(* Logix 5000 AddOnInstructionDefinition export YAI_Assy_166_116_EIP_Hz; software revision 21.03 *)

ADD_ON_INSTRUCTION YAI_Assy_166_116_EIP_Hz   (* revision 1.1, vendor Yaskawa America, Inc. *)
// YAI Assembly 166 and 116
// Revision note:
// Corrected Custom_Out_x function.
// Help:
// This add-on instruction is for use with input assemblie 166 and output assemblies 116.
// Node_Input_Assy is defined as the node's input assembly integer array.
// Node_Output_Assy is defined as the node's output assembly integer array.
// Torque limit/reference, torque compensation and torque output variables are only available with A1000.
VAR_IN_OUT
   Node_Input_Assy : AB:ETHERNET_MODULE_INT_44Bytes:I:0; {required}   // Input assembly words
   Node_Output_Assy : AB:ETHERNET_MODULE_INT_44Bytes:O:0; {required}   // Output assembly words
END_VAR
VAR_INPUT
   RunFwd : BOOL; {visible}   // Forward run command
   RunRev : BOOL; {visible}   // Reverse run command
   MFI_3 : BOOL; {visible}   // Multi-function input 3
   MFI_4 : BOOL; {visible}   // Multi-function input 4
   MFI_5 : BOOL; {visible}   // Multi-function input 5
   MFI_6 : BOOL; {visible}   // Multi-function input 6
   MFI_7 : BOOL; {visible}   // Multi-function input 7
   MFI_8 : BOOL; {visible}   // Multi-function input 8
   External_Fault : BOOL;   // External fault command (EF0)
   FaultReset : BOOL; {visible}   // Fault reset command
   MFO_1 : BOOL; {visible}   // Multi-function output (M1-M2 for A/P1000, MA/MB/MC for V1000)
   MFO_2 : BOOL; {visible}   // Multi-function output (M3-M4 for A/P1000, P1 for V1000)
   MFO_3 : BOOL; {visible}   // Multi-function output (M5-M6 for A/P1000, P2 for V1000)
   Freq_Ref : REAL; {visible}   // Frequency reference command in Hz (xx.xx resolution)
   Torq_Ref_Limit : REAL; {visible}   // Torque reference/limit (A1000 only)
   Torq_Comp : REAL; {visible}   // Torque compensation command (A1000 only)
   Net_Ref : BOOL;   // Network reference control bit
   Net_Control : BOOL;   // Network start/stop control bit
   Analog_Output_1 : REAL;   // Analog output 1 level command
   Analog_Output_2 : REAL;   // Analog output 2 level command
   Digital_Output_1 : BOOL;   // Digital output 1 activation - M1-M2
   Digital_Output_2 : BOOL;   // Digital output 2 activation - M3-M4
   Digital_Output_3 : BOOL;   // Digital output 3 activation - M5-M6
   Digital_Output_Fault_Enable : BOOL;   // Bit to enable control of fault output relay over the network
   Digital_Output_Fault : BOOL;   // Fault relay activation - MA-MB-MC
   Custom_Out_1 : INT; {visible}   // Custom output 1 - F7-23
   Custom_Out_2 : INT; {visible}   // Custom output 2 - F7-24
   Custom_Out_3 : INT; {visible}   // Custom output 3 - F7-25
   Custom_Out_4 : INT;   // Custom output 4 - F7-26
   Custom_Out_5 : INT;   // Custom output 5 - F7-27
   Custom_Out_6 : INT;   // Custom output 6 - F7-28
   Custom_Out_7 : INT;   // Custom output 7 - F7-29
   Custom_Out_8 : INT;   // Custom output 8 - F7-30
   Custom_Out_9 : INT;   // Custom output 9 - F7-31
   Custom_Out_10 : INT;   // Custom output 10 - F7-32
END_VAR
VAR_OUTPUT
   Running : BOOL; {access Read Only, visible}   // Drive running forward status bit
   ZSP : BOOL; {access Read Only, visible}   // Drive zero speed status bit
   RunningRev : BOOL; {access Read Only, visible}   // Drive running reverse status bit
   Reset : BOOL; {access Read Only, visible}   // Drive reset command status bit
   At_Speed : BOOL; {access Read Only, visible}   // Drive at commanded speed status bit
   Ready : BOOL; {access Read Only, visible}   // Drive ready status bit
   Alarm : BOOL; {access Read Only, visible}   // Drive alarm status bit
   Faulted : BOOL; {access Read Only, visible}   // Drive faulted status bit
   OPE : BOOL; {access Read Only}   // OPE alarm/fault present
   UV : BOOL; {access Read Only}   // Drive in UV (undervoltage) state status bit
   NetCtrlStatus : BOOL; {access Read Only, visible}   // Drive network run source status bit (1 = source coming from network)
   MFO_1_Status : BOOL; {access Read Only, visible}   // Drive multi-function output 1 (M1-M2 for A/P1000, MA/MB/MC for V1000) status
   MFO_2_Status : BOOL; {access Read Only, visible}   // Drive multi-function output 1 (M3-M4 for A/P1000, P1 for V1000) status
   MFO_3_Status : BOOL; {access Read Only, visible}   // Drive multi-function output 1 (M5-M6 for A/P1000, P2 for V1000) status
   ZSV : BOOL; {access Read Only, visible}   // Drive zero servo completed status bit
   Motor_Speed : REAL; {access Read Only, visible}   // Motor speed in Hz (xx.xx resolution)
   Torque_Actual : REAL; {access Read Only, visible}   // Drive torque output in % (xxx.x resolution)
   PG_Count : INT; {access Read Only}   // Encoder feedback count
   Freq_Cmd : REAL; {access Read Only, visible}   // Commanded frequency in Hz (xx.xx resolution)
   Output_Freq : REAL; {access Read Only, visible}   // Drive output frequency in Hz (xx.xx resolution)
   Output_Current : REAL; {access Read Only, visible}   // Drive output current in A (xxx.x resolution)
   Analog_Input_1_Level : REAL; {access Read Only}   // Analog input 1 level in % (xxx.x resolution)
   DC_Bus_Volt : INT; {access Read Only, visible}   // DC bus voltage in Vdc (xxx resolution)
   Error_Code : INT; {access Read Only}   // Custom input/output error code. Refer to custom error bit to determine which parameter error is pertaining to.
   Custom_In_1 : INT; {access Read Only, visible}   // Custom input 1 - F7-33
   Custom_In_2 : INT; {access Read Only, visible}   // Custom input 2 - F7-34
   Custom_In_3 : INT; {access Read Only, visible}   // Custom input 3 - F7-35
   Custom_In_4 : INT; {access Read Only}   // Custom input 4 - F7-36
   Custom_In_5 : INT; {access Read Only}   // Custom input 5 - F7-37
   Custom_In_6 : INT; {access Read Only}   // Custom input 6 - F7-38
   Custom_In_7 : INT; {access Read Only}   // Custom input 7 - F7-39
   Custom_In_8 : INT; {access Read Only}   // Custom input 8 -F7-40
   Custom_In_9 : INT; {access Read Only}   // Custom input 9 - F7-41
   Custom_In_10 : INT; {access Read Only}   // Custom input 10 - F7-42
   Custom_Out_1_Error : BOOL; {access Read Only}   // Custom output 1 error bit
   Custom_Out_2_Error : BOOL; {access Read Only}   // Custom output 2 error bit
   Custom_Out_3_Error : BOOL; {access Read Only}   // Custom output 3 error bit
   Custom_Out_4_Error : BOOL; {access Read Only}   // Custom output 4 error bit
   Custom_Out_5_Error : BOOL; {access Read Only}   // Custom output 5 error bit
   Custom_Out_6_Error : BOOL; {access Read Only}   // Custom output 6 error bit
   Custom_Out_7_Error : BOOL; {access Read Only}   // Custom output 7 error bit
   Custom_Out_8_Error : BOOL; {access Read Only}   // Custom output 8 error bit
   Custom_Out_9_Error : BOOL; {access Read Only}   // Custom output 9 error bit
   Custom_Out_10_Error : BOOL; {access Read Only}   // Custom output 10 error bit
   Custom_In_1_Error : BOOL; {access Read Only}   // Custom input 1 error bit
   Custom_In_2_Error : BOOL; {access Read Only}   // Custom input 2 error bit
   Custom_In_3_Error : BOOL; {access Read Only}   // Custom input 3 error bit
   Custom_In_4_Error : BOOL; {access Read Only}   // Custom input 4 error bit
   Custom_In_5_Error : BOOL; {access Read Only}   // Custom input 5 error bit
   Custom_In_6_Error : BOOL; {access Read Only}   // Custom input 6 error bit
   Custom_In_7_Error : BOOL; {access Read Only}   // Custom input 7 error bit
   Custom_In_8_Error : BOOL; {access Read Only}   // Custom input 8 error bit
   Custom_In_9_Error : BOOL; {access Read Only}   // Custom input 9 error bit
   Custom_In_10_Error : BOOL; {access Read Only}   // Custom input 10 error bit
END_VAR
VAR
   FRef_Convert : DINT;
   FOut_Convert : REAL;
   FOut_Temp : REAL;
   TRef_Convert : INT;
   TComp_Convert : INT;
   TOut_Convert : REAL;
   TOut_Temp : REAL;
   IOut_Temp : REAL;
   IOut_Convert : REAL;
   AO1_Convert : INT;
   AO2_Convert : INT;
   Motor_Speed_Temp : REAL;
   Motor_Speed_Convert : REAL;
   Freq_Cmd_Temp : REAL;
   Freq_Cmd_Convert : REAL;
   AI1_Temp : REAL;
   AI1_Convert : REAL;
END_VAR

ROUTINE Logic   (* ladder *)
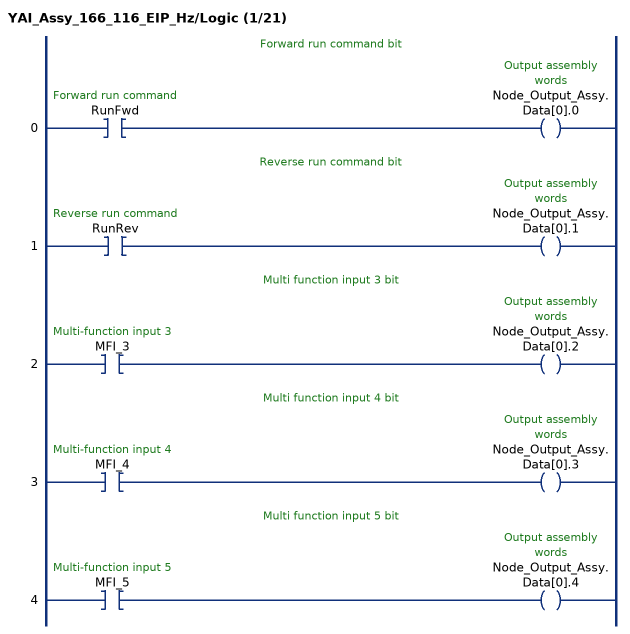
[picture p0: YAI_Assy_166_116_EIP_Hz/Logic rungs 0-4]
   // Forward run command bit
   0: XIC(RunFwd)OTE(Node_Output_Assy.Data[0].0);
   // Reverse run command bit
   1: XIC(RunRev)OTE(Node_Output_Assy.Data[0].1);
   // Multi function input 3 bit
   2: XIC(MFI_3)OTE(Node_Output_Assy.Data[0].2);
   // Multi function input 4 bit
   3: XIC(MFI_4)OTE(Node_Output_Assy.Data[0].3);
   // Multi function input 5 bit
   4: XIC(MFI_5)OTE(Node_Output_Assy.Data[0].4);
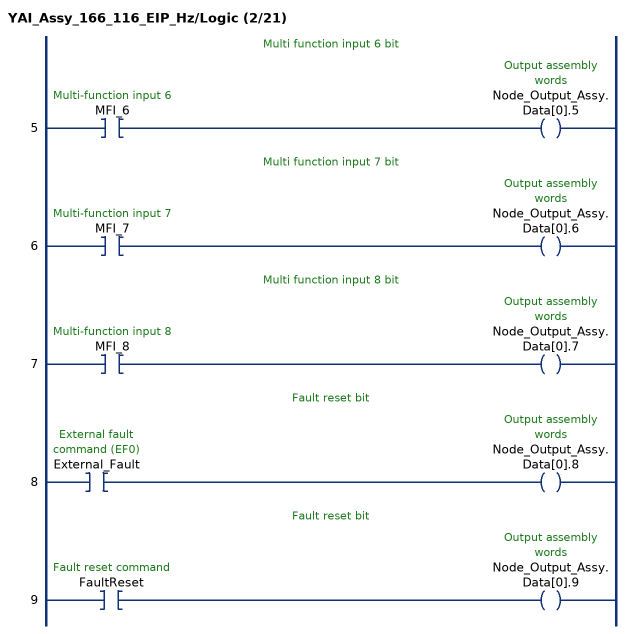
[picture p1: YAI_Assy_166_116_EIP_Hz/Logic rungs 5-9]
   // Multi function input 6 bit
   5: XIC(MFI_6)OTE(Node_Output_Assy.Data[0].5);
   // Multi function input 7 bit
   6: XIC(MFI_7)OTE(Node_Output_Assy.Data[0].6);
   // Multi function input 8 bit
   7: XIC(MFI_8)OTE(Node_Output_Assy.Data[0].7);
   // Fault reset bit
   8: XIC(External_Fault)OTE(Node_Output_Assy.Data[0].8);
   // Fault reset bit
   9: XIC(FaultReset)OTE(Node_Output_Assy.Data[0].9);
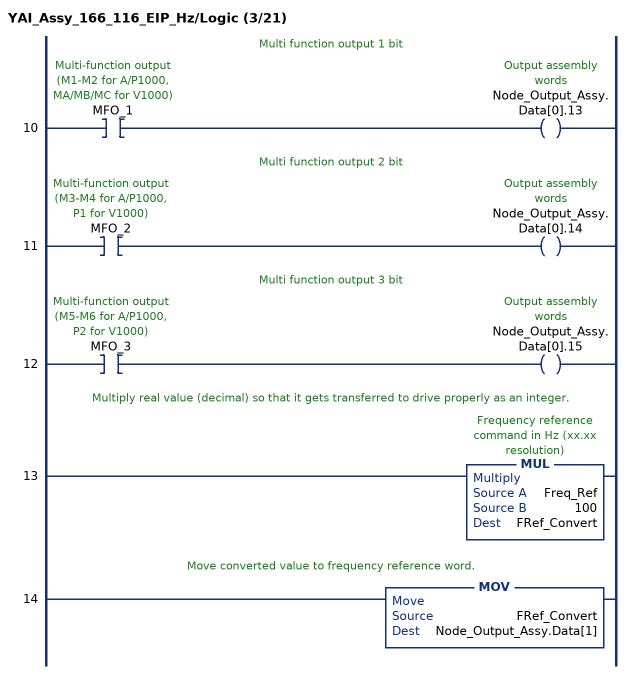
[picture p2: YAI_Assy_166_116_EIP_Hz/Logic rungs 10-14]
   // Multi function output 1 bit
   10: XIC(MFO_1)OTE(Node_Output_Assy.Data[0].13);
   // Multi function output 2 bit
   11: XIC(MFO_2)OTE(Node_Output_Assy.Data[0].14);
   // Multi function output 3 bit
   12: XIC(MFO_3)OTE(Node_Output_Assy.Data[0].15);
   // Multiply real value (decimal) so that it gets transferred to drive properly as an integer.
   13: MUL(Freq_Ref,100,FRef_Convert);
   // Move converted value to frequency reference word.
   14: MOV(FRef_Convert,Node_Output_Assy.Data[1]);
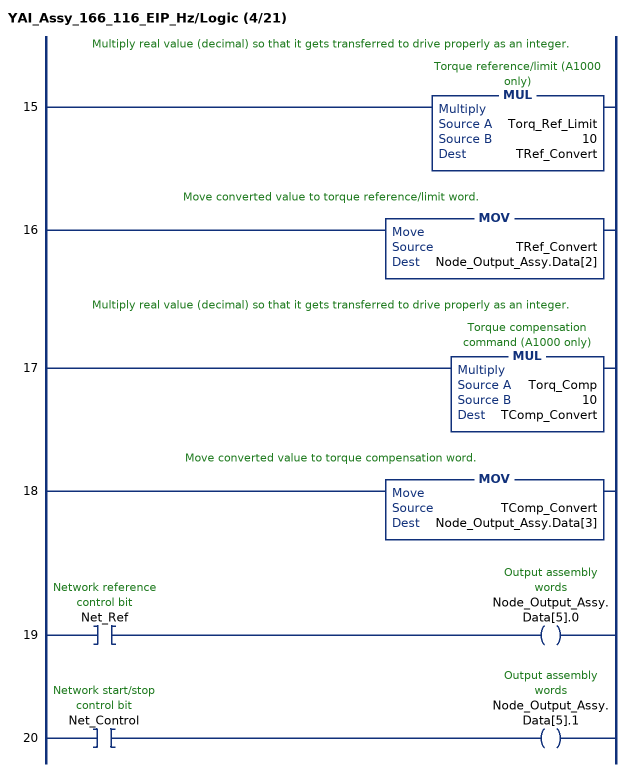
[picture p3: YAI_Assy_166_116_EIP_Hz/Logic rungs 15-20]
   // Multiply real value (decimal) so that it gets transferred to drive properly as an integer.
   15: MUL(Torq_Ref_Limit,10,TRef_Convert);
   // Move converted value to torque reference/limit word.
   16: MOV(TRef_Convert,Node_Output_Assy.Data[2]);
   // Multiply real value (decimal) so that it gets transferred to drive properly as an integer.
   17: MUL(Torq_Comp,10,TComp_Convert);
   // Move converted value to torque compensation word.
   18: MOV(TComp_Convert,Node_Output_Assy.Data[3]);
   19: XIC(Net_Ref)OTE(Node_Output_Assy.Data[5].0);
   20: XIC(Net_Control)OTE(Node_Output_Assy.Data[5].1);
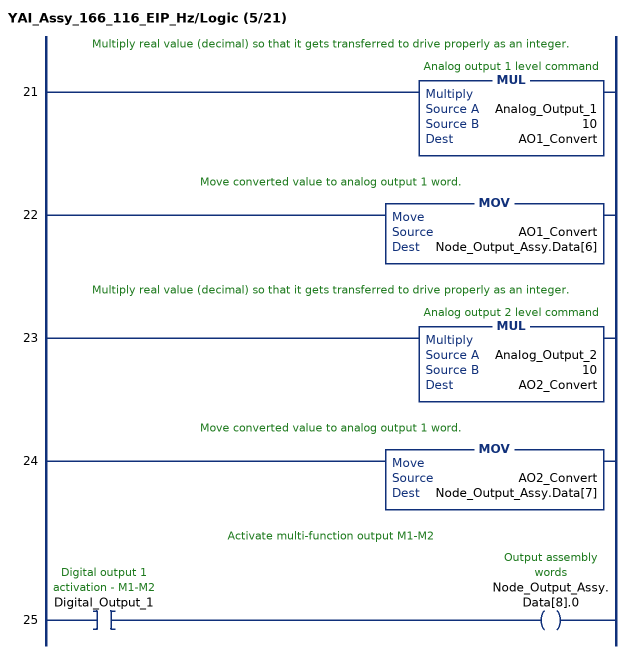
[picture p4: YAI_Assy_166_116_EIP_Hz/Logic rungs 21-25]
   // Multiply real value (decimal) so that it gets transferred to drive properly as an integer.
   21: MUL(Analog_Output_1,10,AO1_Convert);
   // Move converted value to analog output 1 word.
   22: MOV(AO1_Convert,Node_Output_Assy.Data[6]);
   // Multiply real value (decimal) so that it gets transferred to drive properly as an integer.
   23: MUL(Analog_Output_2,10,AO2_Convert);
   // Move converted value to analog output 1 word.
   24: MOV(AO2_Convert,Node_Output_Assy.Data[7]);
   // Activate multi-function output M1-M2
   25: XIC(Digital_Output_1)OTE(Node_Output_Assy.Data[8].0);
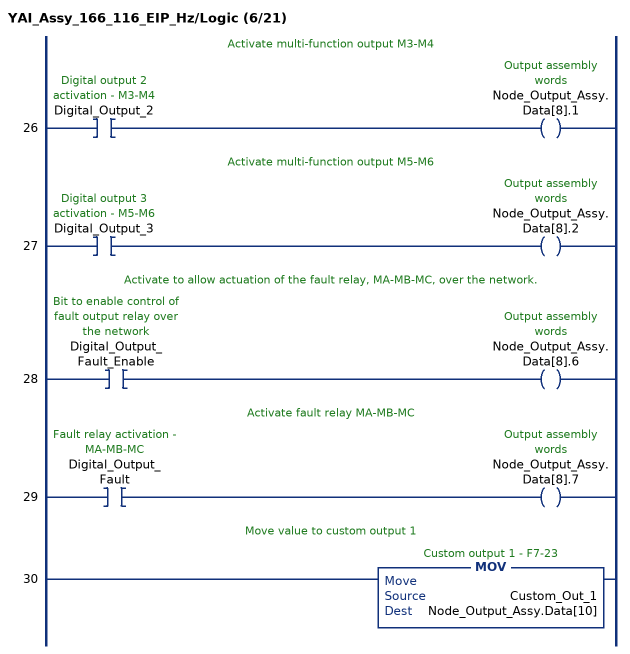
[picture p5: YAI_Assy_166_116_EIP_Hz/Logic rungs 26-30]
   // Activate multi-function output M3-M4
   26: XIC(Digital_Output_2)OTE(Node_Output_Assy.Data[8].1);
   // Activate multi-function output M5-M6
   27: XIC(Digital_Output_3)OTE(Node_Output_Assy.Data[8].2);
   // Activate to allow actuation of the fault relay, MA-MB-MC, over the network.
   28: XIC(Digital_Output_Fault_Enable)OTE(Node_Output_Assy.Data[8].6);
   // Activate fault relay MA-MB-MC
   29: XIC(Digital_Output_Fault)OTE(Node_Output_Assy.Data[8].7);
   // Move value to custom output 1
   30: MOV(Custom_Out_1,Node_Output_Assy.Data[10]);
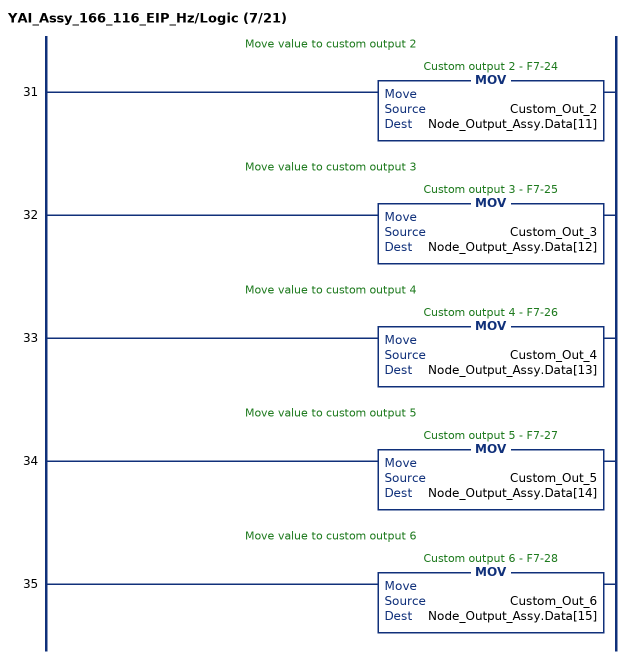
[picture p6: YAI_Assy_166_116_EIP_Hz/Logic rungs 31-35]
   // Move value to custom output 2
   31: MOV(Custom_Out_2,Node_Output_Assy.Data[11]);
   // Move value to custom output 3
   32: MOV(Custom_Out_3,Node_Output_Assy.Data[12]);
   // Move value to custom output 4
   33: MOV(Custom_Out_4,Node_Output_Assy.Data[13]);
   // Move value to custom output 5
   34: MOV(Custom_Out_5,Node_Output_Assy.Data[14]);
   // Move value to custom output 6
   35: MOV(Custom_Out_6,Node_Output_Assy.Data[15]);
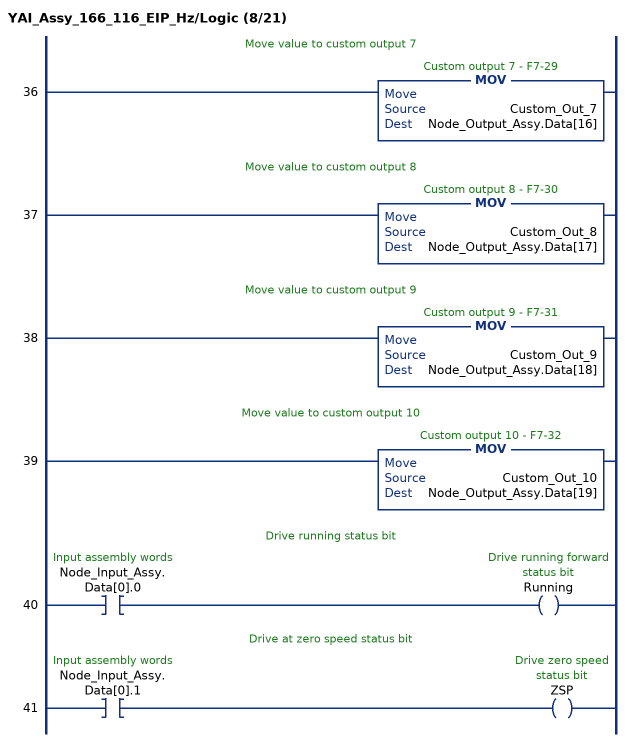
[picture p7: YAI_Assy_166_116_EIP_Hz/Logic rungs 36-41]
   // Move value to custom output 7
   36: MOV(Custom_Out_7,Node_Output_Assy.Data[16]);
   // Move value to custom output 8
   37: MOV(Custom_Out_8,Node_Output_Assy.Data[17]);
   // Move value to custom output 9
   38: MOV(Custom_Out_9,Node_Output_Assy.Data[18]);
   // Move value to custom output 10
   39: MOV(Custom_Out_10,Node_Output_Assy.Data[19]);
   // Drive running status bit
   40: XIC(Node_Input_Assy.Data[0].0)OTE(Running);
   // Drive at zero speed status bit
   41: XIC(Node_Input_Assy.Data[0].1)OTE(ZSP);
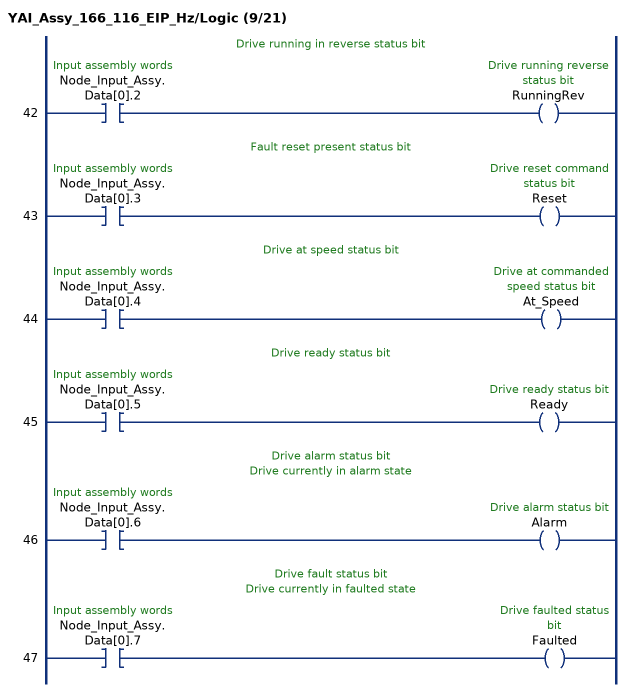
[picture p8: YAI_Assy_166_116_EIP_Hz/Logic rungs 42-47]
   // Drive running in reverse status bit
   42: XIC(Node_Input_Assy.Data[0].2)OTE(RunningRev);
   // Fault reset present status bit
   43: XIC(Node_Input_Assy.Data[0].3)OTE(Reset);
   // Drive at speed status bit
   44: XIC(Node_Input_Assy.Data[0].4)OTE(At_Speed);
   // Drive ready status bit
   45: XIC(Node_Input_Assy.Data[0].5)OTE(Ready);
   // Drive alarm status bit
   // Drive currently in alarm state
   46: XIC(Node_Input_Assy.Data[0].6)OTE(Alarm);
   // Drive fault status bit
   // Drive currently in faulted state
   47: XIC(Node_Input_Assy.Data[0].7)OTE(Faulted);
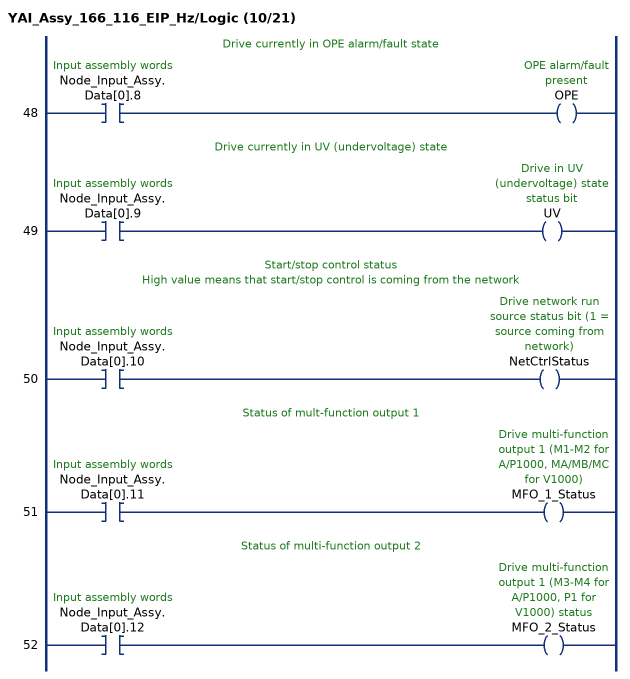
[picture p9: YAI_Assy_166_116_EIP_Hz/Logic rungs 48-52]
   // Drive currently in OPE alarm/fault state
   48: XIC(Node_Input_Assy.Data[0].8)OTE(OPE);
   // Drive currently in UV (undervoltage) state
   49: XIC(Node_Input_Assy.Data[0].9)OTE(UV);
   // Start/stop control status
   // High value means that start/stop control is coming from the network
   50: XIC(Node_Input_Assy.Data[0].10)OTE(NetCtrlStatus);
   // Status of mult-function output 1
   51: XIC(Node_Input_Assy.Data[0].11)OTE(MFO_1_Status);
   // Status of multi-function output 2
   52: XIC(Node_Input_Assy.Data[0].12)OTE(MFO_2_Status);
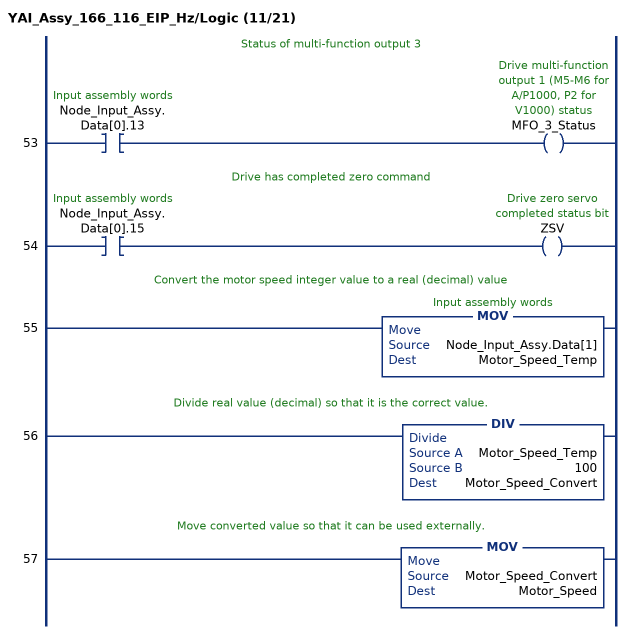
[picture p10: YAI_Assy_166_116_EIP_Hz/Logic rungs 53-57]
   // Status of multi-function output 3
   53: XIC(Node_Input_Assy.Data[0].13)OTE(MFO_3_Status);
   // Drive has completed zero command
   54: XIC(Node_Input_Assy.Data[0].15)OTE(ZSV);
   // Convert the motor speed integer value to a real (decimal) value
   55: MOV(Node_Input_Assy.Data[1],Motor_Speed_Temp);
   // Divide real value (decimal) so that it is the correct value.
   56: DIV(Motor_Speed_Temp,100,Motor_Speed_Convert);
   // Move converted value so that it can be used externally.
   57: MOV(Motor_Speed_Convert,Motor_Speed);
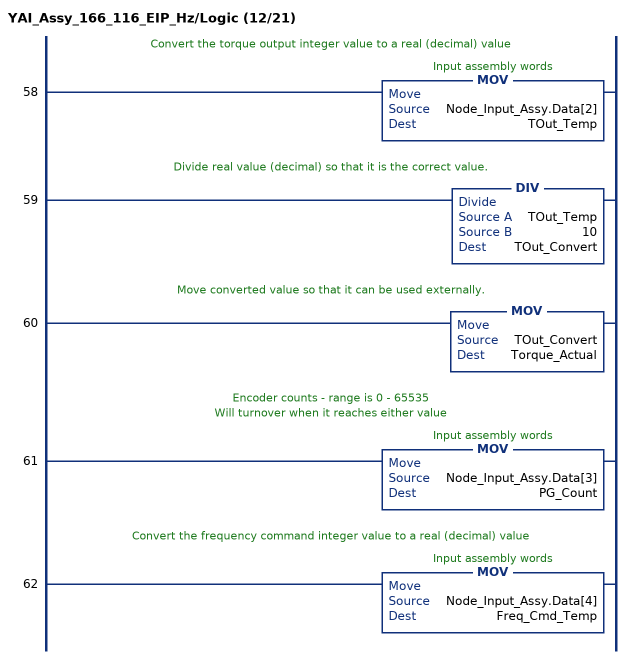
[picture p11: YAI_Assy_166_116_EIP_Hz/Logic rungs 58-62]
   // Convert the torque output integer value to a real (decimal) value
   58: MOV(Node_Input_Assy.Data[2],TOut_Temp);
   // Divide real value (decimal) so that it is the correct value.
   59: DIV(TOut_Temp,10,TOut_Convert);
   // Move converted value so that it can be used externally.
   60: MOV(TOut_Convert,Torque_Actual);
   // Encoder counts - range is 0 - 65535
   // Will turnover when it reaches either value
   61: MOV(Node_Input_Assy.Data[3],PG_Count);
   // Convert the frequency command integer value to a real (decimal) value
   62: MOV(Node_Input_Assy.Data[4],Freq_Cmd_Temp);
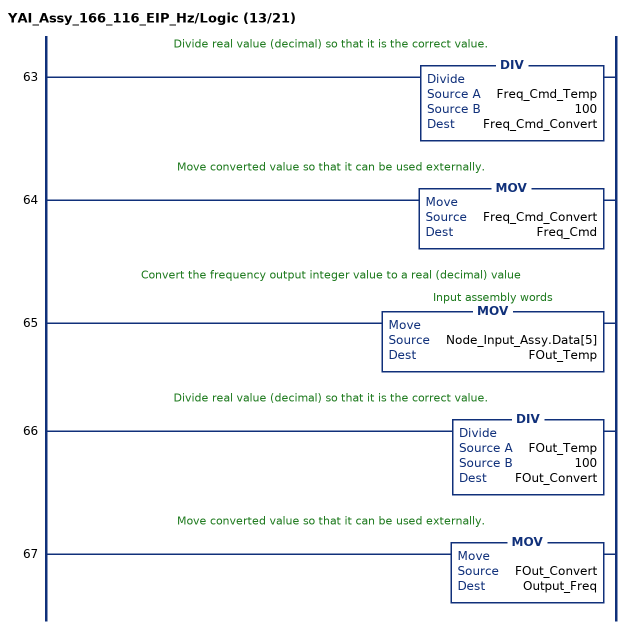
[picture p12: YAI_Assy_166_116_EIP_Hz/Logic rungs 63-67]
   // Divide real value (decimal) so that it is the correct value.
   63: DIV(Freq_Cmd_Temp,100,Freq_Cmd_Convert);
   // Move converted value so that it can be used externally.
   64: MOV(Freq_Cmd_Convert,Freq_Cmd);
   // Convert the frequency output integer value to a real (decimal) value
   65: MOV(Node_Input_Assy.Data[5],FOut_Temp);
   // Divide real value (decimal) so that it is the correct value.
   66: DIV(FOut_Temp,100,FOut_Convert);
   // Move converted value so that it can be used externally.
   67: MOV(FOut_Convert,Output_Freq);
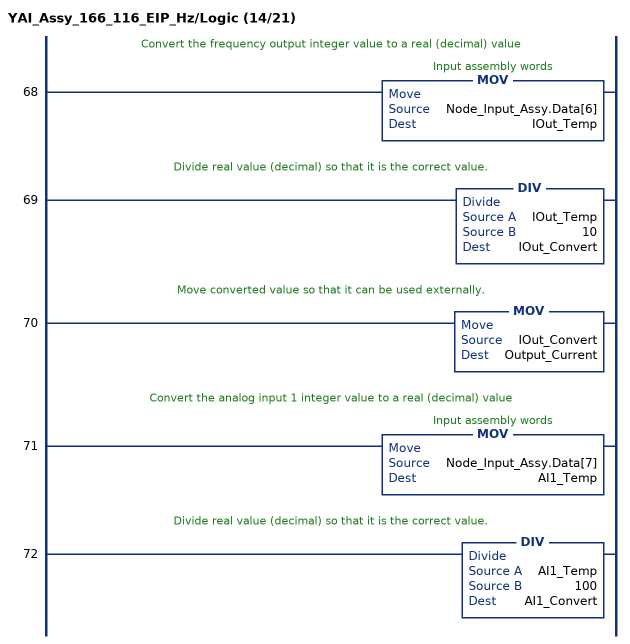
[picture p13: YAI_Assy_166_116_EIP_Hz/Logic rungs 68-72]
   // Convert the frequency output integer value to a real (decimal) value
   68: MOV(Node_Input_Assy.Data[6],IOut_Temp);
   // Divide real value (decimal) so that it is the correct value.
   69: DIV(IOut_Temp,10,IOut_Convert);
   // Move converted value so that it can be used externally.
   70: MOV(IOut_Convert,Output_Current);
   // Convert the analog input 1 integer value to a real (decimal) value
   71: MOV(Node_Input_Assy.Data[7],AI1_Temp);
   // Divide real value (decimal) so that it is the correct value.
   72: DIV(AI1_Temp,100,AI1_Convert);
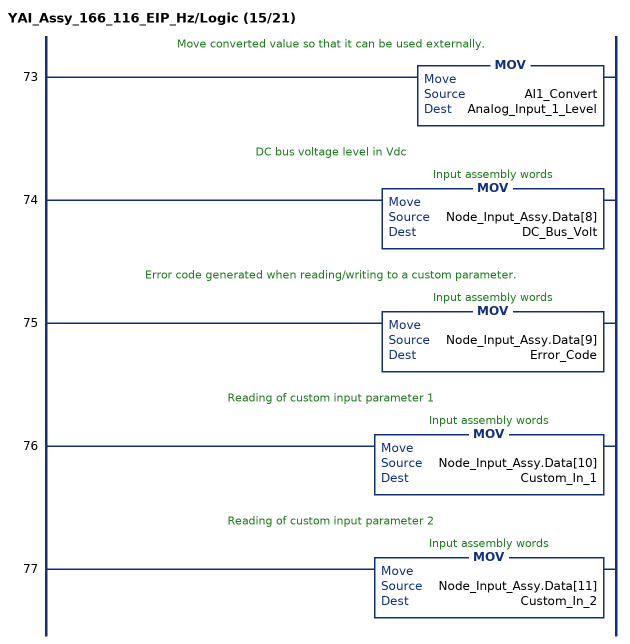
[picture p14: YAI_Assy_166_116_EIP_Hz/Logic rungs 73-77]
   // Move converted value so that it can be used externally.
   73: MOV(AI1_Convert,Analog_Input_1_Level);
   // DC bus voltage level in Vdc
   74: MOV(Node_Input_Assy.Data[8],DC_Bus_Volt);
   // Error code generated when reading/writing to a custom parameter.
   75: MOV(Node_Input_Assy.Data[9],Error_Code);
   // Reading of custom input parameter 1
   76: MOV(Node_Input_Assy.Data[10],Custom_In_1);
   // Reading of custom input parameter 2
   77: MOV(Node_Input_Assy.Data[11],Custom_In_2);
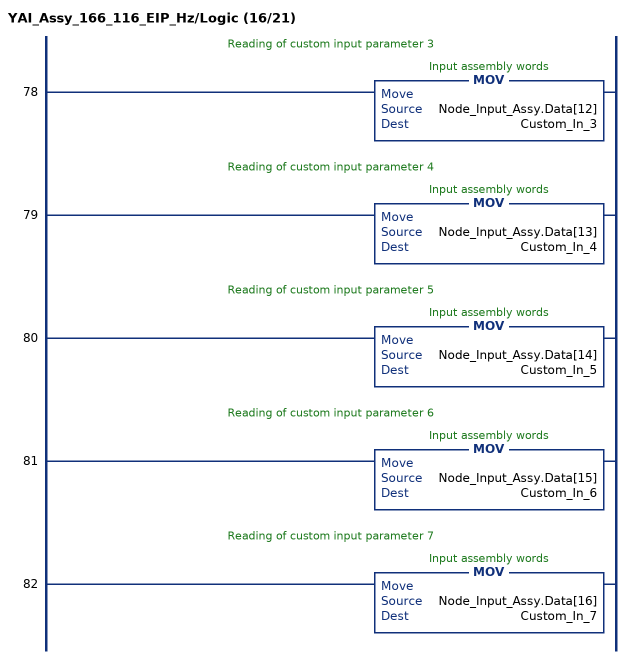
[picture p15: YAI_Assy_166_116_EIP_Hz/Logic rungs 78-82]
   // Reading of custom input parameter 3
   78: MOV(Node_Input_Assy.Data[12],Custom_In_3);
   // Reading of custom input parameter 4
   79: MOV(Node_Input_Assy.Data[13],Custom_In_4);
   // Reading of custom input parameter 5
   80: MOV(Node_Input_Assy.Data[14],Custom_In_5);
   // Reading of custom input parameter 6
   81: MOV(Node_Input_Assy.Data[15],Custom_In_6);
   // Reading of custom input parameter 7
   82: MOV(Node_Input_Assy.Data[16],Custom_In_7);
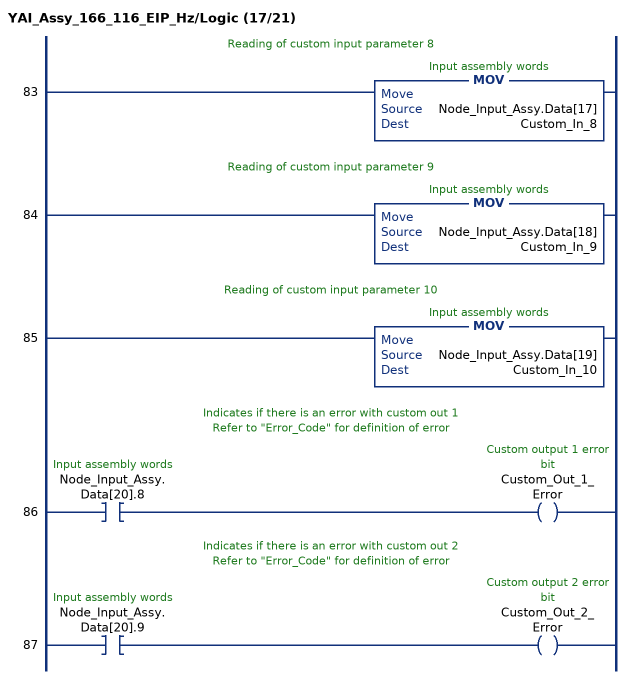
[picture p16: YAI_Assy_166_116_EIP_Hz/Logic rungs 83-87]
   // Reading of custom input parameter 8
   83: MOV(Node_Input_Assy.Data[17],Custom_In_8);
   // Reading of custom input parameter 9
   84: MOV(Node_Input_Assy.Data[18],Custom_In_9);
   // Reading of custom input parameter 10
   85: MOV(Node_Input_Assy.Data[19],Custom_In_10);
   // Indicates if there is an error with custom out 1
   // Refer to "Error_Code" for definition of error
   86: XIC(Node_Input_Assy.Data[20].8)OTE(Custom_Out_1_Error);
   // Indicates if there is an error with custom out 2
   // Refer to "Error_Code" for definition of error
   87: XIC(Node_Input_Assy.Data[20].9)OTE(Custom_Out_2_Error);
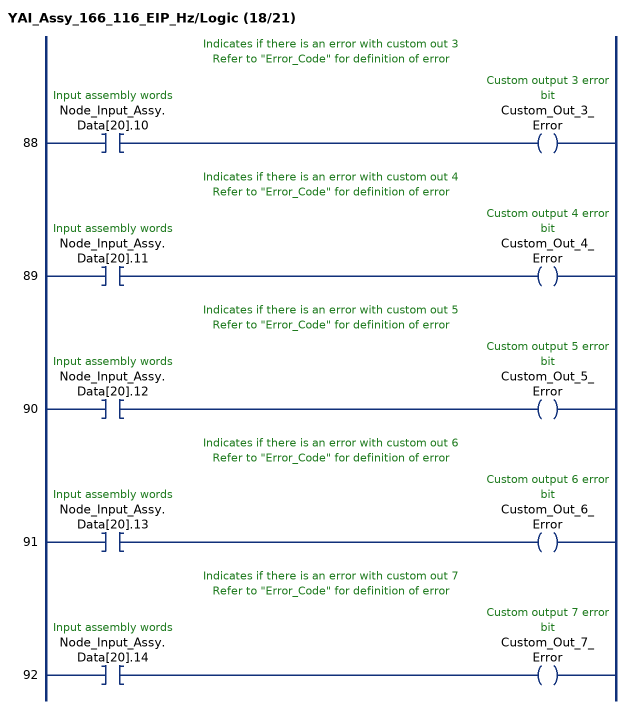
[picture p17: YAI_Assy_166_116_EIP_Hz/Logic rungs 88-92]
   // Indicates if there is an error with custom out 3
   // Refer to "Error_Code" for definition of error
   88: XIC(Node_Input_Assy.Data[20].10)OTE(Custom_Out_3_Error);
   // Indicates if there is an error with custom out 4
   // Refer to "Error_Code" for definition of error
   89: XIC(Node_Input_Assy.Data[20].11)OTE(Custom_Out_4_Error);
   // Indicates if there is an error with custom out 5
   // Refer to "Error_Code" for definition of error
   90: XIC(Node_Input_Assy.Data[20].12)OTE(Custom_Out_5_Error);
   // Indicates if there is an error with custom out 6
   // Refer to "Error_Code" for definition of error
   91: XIC(Node_Input_Assy.Data[20].13)OTE(Custom_Out_6_Error);
   // Indicates if there is an error with custom out 7
   // Refer to "Error_Code" for definition of error
   92: XIC(Node_Input_Assy.Data[20].14)OTE(Custom_Out_7_Error);
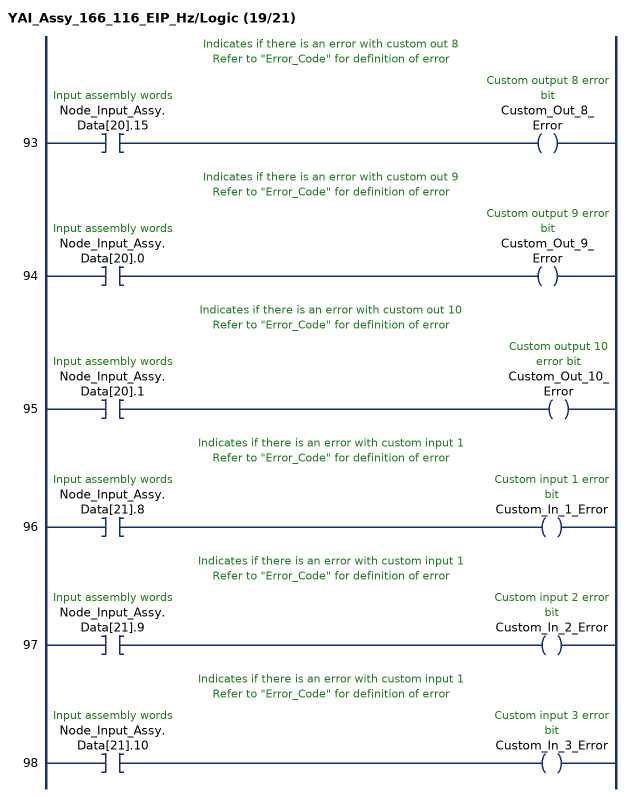
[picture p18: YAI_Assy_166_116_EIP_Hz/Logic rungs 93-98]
   // Indicates if there is an error with custom out 8
   // Refer to "Error_Code" for definition of error
   93: XIC(Node_Input_Assy.Data[20].15)OTE(Custom_Out_8_Error);
   // Indicates if there is an error with custom out 9
   // Refer to "Error_Code" for definition of error
   94: XIC(Node_Input_Assy.Data[20].0)OTE(Custom_Out_9_Error);
   // Indicates if there is an error with custom out 10
   // Refer to "Error_Code" for definition of error
   95: XIC(Node_Input_Assy.Data[20].1)OTE(Custom_Out_10_Error);
   // Indicates if there is an error with custom input 1
   // Refer to "Error_Code" for definition of error
   96: XIC(Node_Input_Assy.Data[21].8)OTE(Custom_In_1_Error);
   // Indicates if there is an error with custom input 1
   // Refer to "Error_Code" for definition of error
   97: XIC(Node_Input_Assy.Data[21].9)OTE(Custom_In_2_Error);
   // Indicates if there is an error with custom input 1
   // Refer to "Error_Code" for definition of error
   98: XIC(Node_Input_Assy.Data[21].10)OTE(Custom_In_3_Error);
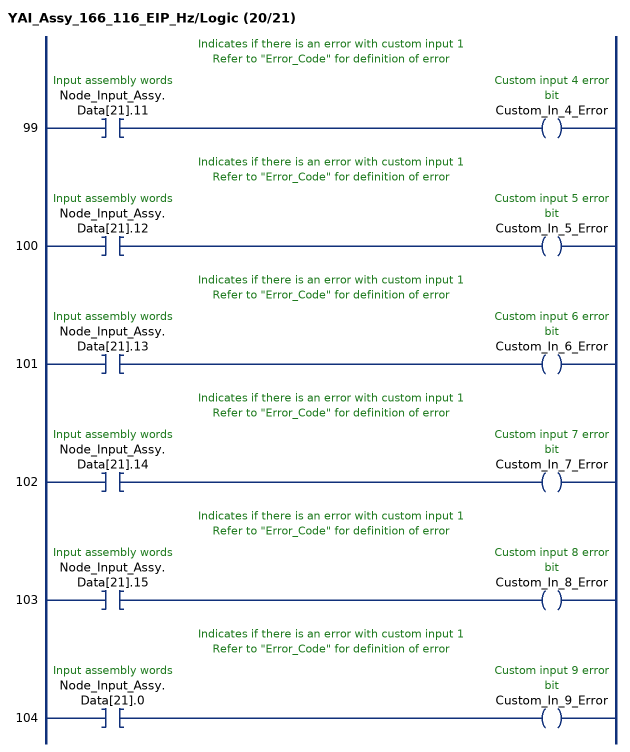
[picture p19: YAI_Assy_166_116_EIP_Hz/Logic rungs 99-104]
   // Indicates if there is an error with custom input 1
   // Refer to "Error_Code" for definition of error
   99: XIC(Node_Input_Assy.Data[21].11)OTE(Custom_In_4_Error);
   // Indicates if there is an error with custom input 1
   // Refer to "Error_Code" for definition of error
   100: XIC(Node_Input_Assy.Data[21].12)OTE(Custom_In_5_Error);
   // Indicates if there is an error with custom input 1
   // Refer to "Error_Code" for definition of error
   101: XIC(Node_Input_Assy.Data[21].13)OTE(Custom_In_6_Error);
   // Indicates if there is an error with custom input 1
   // Refer to "Error_Code" for definition of error
   102: XIC(Node_Input_Assy.Data[21].14)OTE(Custom_In_7_Error);
   // Indicates if there is an error with custom input 1
   // Refer to "Error_Code" for definition of error
   103: XIC(Node_Input_Assy.Data[21].15)OTE(Custom_In_8_Error);
   // Indicates if there is an error with custom input 1
   // Refer to "Error_Code" for definition of error
   104: XIC(Node_Input_Assy.Data[21].0)OTE(Custom_In_9_Error);
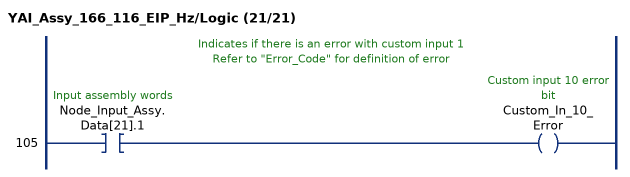
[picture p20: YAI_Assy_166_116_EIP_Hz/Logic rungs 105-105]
   // Indicates if there is an error with custom input 1
   // Refer to "Error_Code" for definition of error
   105: XIC(Node_Input_Assy.Data[21].1)OTE(Custom_In_10_Error);
END_ROUTINE
END_ADD_ON_INSTRUCTION
